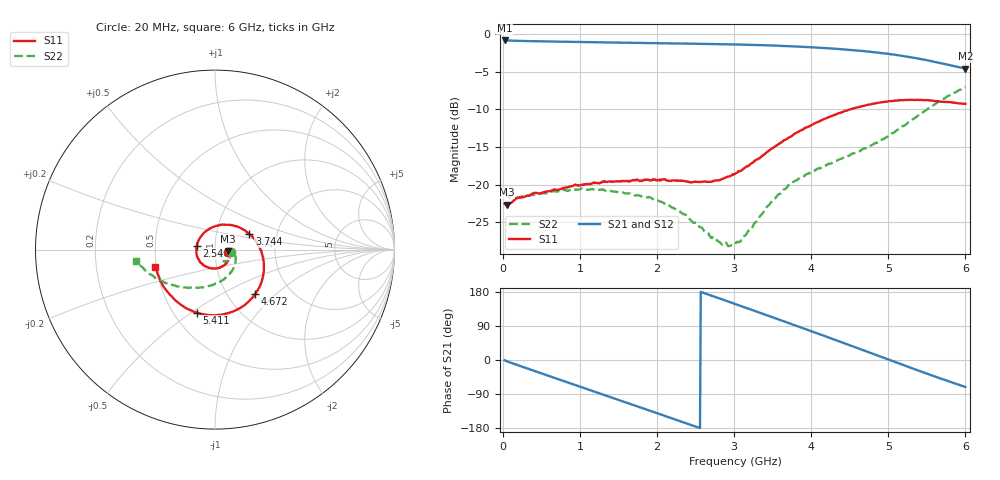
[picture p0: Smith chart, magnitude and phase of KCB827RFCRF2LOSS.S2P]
!Agilent Technologies,E5071B,JP1KK00126,A.08.11
!Date: Tue May 06 07:26:49 2014
!Data & Calibration Information:
!Freq	S11:SOLT2(ON)	S21:SOLT2(ON)	S12:SOLT2(ON)	S22:SOLT2(ON)
# Hz S dB R 50
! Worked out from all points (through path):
!   600 points, 20 MHz to 6 GHz, reference 50 ohm
!   highest |S21| = -0.83 dB at 20 MHz (marker M1); lowest = -4.6 dB at 6 GHz (marker M2)
!   group delay of S21, straight-line fit = 200 ps
!   lowest |S11| = -22.7 dB at 49.95 MHz (marker M3), VSWR 1.16, Z = 57.9 - j0.953 ohm
!   |S11| at or under -10 dB: start of sweep to 4.503 GHz
!   |S22| runs from -28.2 to -7.0 dB; largest |S21 - S12| = 0.0049
!   S11 on the Smith chart (normalised r, x): 20 MHz: 1.16, -0.04; 2.546 GHz: 0.81, +0.03; 3.744 GHz: 1.45, +0.26; 4.672 GHz: 1.34, -0.74; 5.411 GHz: 0.65, -0.53; 6 GHz: 0.49, -0.11
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2e7  -22.52 -12.3  -0.83 -0.7  -0.82 -0.7  -21.06 -9.6
4.994992e7  -22.66 -6.4  -0.84 -3.4  -0.83 -3.4  -21.37 -4.6
4.991987e8  -21.09 -23.2  -0.95 -35.4  -0.95 -35.4  -21.13 -12.1
7.587646e8  -20.53 -38.6  -1.00 -53.7  -1.00 -53.7  -20.71 -20.5
1.018331e9  -20.02 -55.2  -1.04 -71.7  -1.04 -71.8  -20.49 -28.2
1.247947e9  -19.83 -72.0  -1.08 -87.8  -1.07 -87.8  -20.69 -35.7
1.497529e9  -19.56 -90.3  -1.12 -105.3  -1.11 -105.2  -21.01 -43.0
1.747112e9  -19.38 -109.7  -1.15 -122.7  -1.16 -122.8  -21.40 -49.7
2.016661e9  -19.43 -133.2  -1.21 -141.7  -1.21 -141.7  -22.14 -54.3
2.28621e9  -19.48 -160.5  -1.25 -160.7  -1.25 -160.7  -23.50 -55.8
2.545776e9  -19.63 168.8  -1.28 -179.0  -1.29 -179.0  -25.56 -53.1
2.835292e9  -19.27 130.9  -1.33 160.4  -1.33 160.4  -27.88 -37.9
3.014992e9  -18.53 107.5  -1.36 147.6  -1.37 147.5  -27.82 -22.8
3.394357e9  -15.95 59.6  -1.46 120.2  -1.47 120.1  -23.37 0.1
3.743773e9  -13.55 24.1  -1.60 94.7  -1.61 94.7  -19.92 -5.5
4.013322e9  -12.02 1.4  -1.74 75.0  -1.75 74.9  -18.21 -19.7
4.362738e9  -10.48 -24.9  -1.97 49.1  -1.97 49.0  -16.65 -46.0
4.67222e9  -9.56 -47.7  -2.24 26.0  -2.24 25.9  -15.23 -72.9
5.011653e9  -8.90 -72.6  -2.63 0.5  -2.62 0.4  -13.44 -104.2
5.410985e9  -8.74 -105.9  -3.28 -29.4  -3.27 -29.5  -10.59 -136.0
5.710484e9  -8.98 -134.6  -3.92 -51.0  -3.91 -51.2  -8.62 -155.5
6e9  -9.24 -164.1  -4.57 -71.2  -4.57 -71.2  -7.03 -172.1
